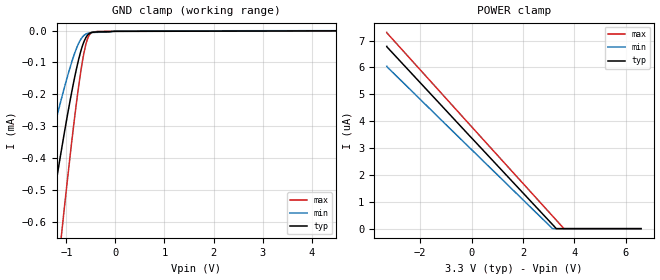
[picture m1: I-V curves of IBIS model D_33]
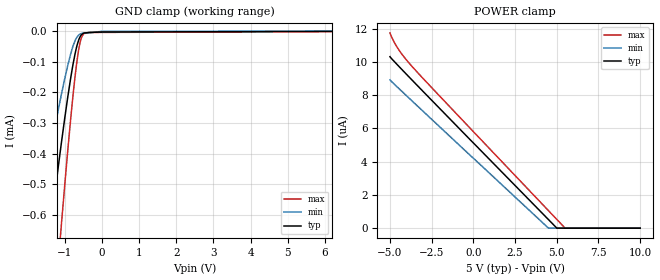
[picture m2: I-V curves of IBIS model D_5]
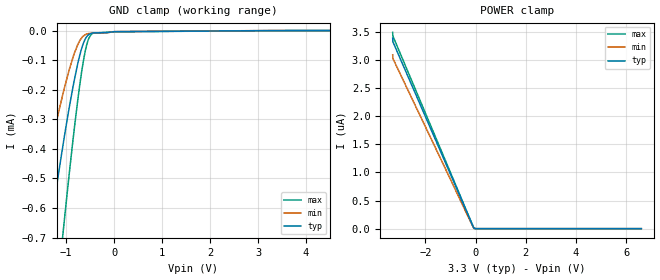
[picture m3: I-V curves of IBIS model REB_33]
| Texas Instruments Incorporated
| Isolated 5-V Full Duplex RS-485 Transceiver
| Bit Rate of 20 Mbps
| Marketing part#   Voltage Range   Package-type   #pins/pkg drawing
| ISO3086DW   3.15V - 5.5V   R-PSOP-G16   16-pin DW
[IBIS Ver]   4.1
[File name]   iso3086e.ibs
[File Rev]   1.0
[Date]   05/04/2010
[Source]   Model built from TISPICE simulations at:
   Texas Instruments Incorporated.
   Analog-eLab, HPA
   12500 TI Blvd
   Dallas, TX -75243
   For Support e-mail: elab_scm_ibis@list.ti.com
[Notes]   Revision History
   Rev 1.0: 05/04/2010
   - Model based on simulations from TIspice
   - Based on simulations, C_comp_typ was lower that C_comp_min
   for pins R, Y and Z
[Disclaimer] This product is designed as an aid for customers of Texas
   Instruments.
   No warranties, either expressed or implied, with respect
   to this third party software (if any) or with respect to
   its fitness for any particular purpose is claimed by Texas
   Instruments or the author. The software (if any) is provided
   solely on an "as is" basis. The entire risk as to its quality
   and performance is with the customer
[Copyright]   (C)Copyright 2010 Texas Instruments Incorporated.
   All rights reserved.
|   Component iso3086e
[Component]   iso3086e
[Manufacturer]  Texas Instruments Incorporated
[Package]   |16-pin PSOP DW package
|   typ   min   max
R_pkg   0.004632   0.00255   0.00893
L_pkg   1.232951nH   0.61490nH   2.36061nH
C_pkg   0.306389pF   0.17825pF   0.45943pF
[Pin] signal_name   model_name   R_pin   L_pin   C_pin
   1  Vcc1   POWER   0.00876   2.29508nH   0.42042pF
   2  GND1   GND   0.00503   1.29566nH   0.28670pF
   3  R   R   0.00282   0.68474nH   0.18911pF
   4  REB   REB   0.00255   0.61553nH   0.17825pF
   5  DE   DE   0.00255   0.61490nH   0.17895pF
   6  D   D   0.00282   0.68226nH   0.19223pF
   7  GND1   GND   0.00276   0.68705nH   0.18198pF
   8  GND1   GND   0.00827   2.24969nH   0.38663pF
   9  GND2   GND   0.00893   2.36061nH   0.43538pF
   10  GND2   GND   0.00586   1.55263nH   0.35752pF
   11  Y   Y   0.00289   0.70650nH   0.19678pF
   12  Z   Z   0.00255   0.61510nH   0.17846pF
   13  B   B   0.00255   0.61510nH   0.17846pF
   14  A   A   0.00289   0.70650nH   0.19678pF
   15  GND2   GND   0.00622   1.64583nH   0.37990pF
   16  Vcc2   POWER   0.00858   2.25489nH   0.45943pF
[Diff_pin]   inv_pin   vdiff   tdelay_typ   tdelay_min   tdelay_max
| The A and B are Diff_pins
| The Y and X are Diff_pins
11   12   0.9   NA   NA   NA
13   14   0.9   NA   NA   NA
[series pin mapping]  pin_2   model_name
4   7   series1M   |REB
5   1   series1M   |DE
6   7   series1M   |D
[Pin Mapping]pulldown_ref pullup_ref gnd_clamp_ref power_clamp_ref |ext_ref
1   NC   PWRBUS1  |Vcc1
2   GNDBUS1   NC   |GND1
3   GNDBUS1   PWRBUS1   NC   NC   | R
4   NC   NC   GNDBUS1   PWRBUS1  | RE_N
5   NC   NC   GNDBUS1   PWRBUS1  | DE
6   NC   NC   GNDBUS1   PWRBUS1  | D
7   GNDBUS1   NC   |GND1
8   GNDBUS1   NC   |GND1
9   GNDBUS2   NC   |GND2 to Y/Z
10   GNDBUS2   NC   |GND2 to Y/Z
11   GNDBUS2   PWRBUS2   NC   NC   | Y   Diff. Out. P
12   GNDBUS2   PWRBUS2   NC   NC   | Z   Diff. Out. N
13   NC   NC   GNDBUS2   PWRBUS2  | B   Diff. Inp. N
14   NC   NC   GNDBUS2   PWRBUS2  | A   Diff. Inp. P
15   GNDBUS2   NC   |GND2 to Y/Z
16   NC   PWRBUS2  |VCC2 to Y/Z
[Model Selector] series1M
series1M_33   series1M model for 3.15V  - 3.60V
series1M_5   series1M model for 4.50V  - 5.50V
[Model Selector] D
D_33   D Input model for 3.15V  - 3.60V
D_5   D Input model for 4.50V  - 5.50V
[Model Selector] DE
DE_33   DE Input model for 3.15V  - 3.60V
DE_5   DE Input model for 4.50V  - 5.50V
[Model Selector] REB
REB_33   REB Input model for 3.15V  - 3.60V
REB_5   REB Input model for 4.50V  - 5.50V
[Model Selector] R
R_33   R Output model for 3.15V  - 3.60V
R_5   R Output model for 4.50V  - 5.50V
[Model Selector] A
A_33   A Differential Input model for 3.15V  - 3.60V  |positive pin
A_5   A Differential Input model for 4.50V  - 5.50V
[Model Selector] B
B_33   B Differential Input model for 3.15V  - 3.60V  |negative pin
B_5   B Differential Input model for 4.50V  - 5.50V
[Model Selector] Y
Y_33   Y Differential 3-state model for 3.15V  - 3.60V  |positive pin
Y_5   Y Differential 3-state model for 4.50V  - 5.50V
[Model Selector] Z
Z_33   Z Differential 3-state model for 3.15V  - 3.60V  |negative pin
Z_5   Z Differential 3-state model for 4.50V  - 5.50V
|   series1M_33 Model
[Model]   series1M_33
Model_type   Series
C_comp   0pF   0pF   0pF
[Voltage Range]   3.3V   3.15V   3.6V
[Pullup Reference]   3.3V   3.15V   3.6V
|It is pullup   resistor for D and REB
|It is pulldown resistor for DE
[Temperature Range]   40   125   -40
[R series]   1e6   NA   NA
|   series1M_5 Model
[Model]   series1M_5
Model_type   Series
C_comp   0pF   0pF   0pF
[Voltage Range]   5V   4.5V   5.5V
[Pullup Reference]   5V   4.5V   5.5V
|It is pullup   resistor for D and REB
|It is pulldown resistor for DE
[Temperature Range]   40   125   -40
[R series]   1e6   NA   NA
| Models and submodels in the file (18): series1M_33 (Series), series1M_5 (Series), D_33 (Input), D_5 (Input), DE_33 (Input), DE_5 (Input), REB_33 (Input), REB_5 (Input), R_33 (3-state), R_5 (3-state), A_33 (Input), B_33 (Input), A_5 (Input), B_5 (Input), Y_33 (3-state), Z_33 (3-state), Y_5 (3-state), Z_5 (3-state)
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|   D_33 Model
[Model]   D_33
Model_type   Input
Vinl   = 0.8
Vinh   = 2
|   typ   min   max
C_comp   768fF   754fF   769fF
[Voltage Range]   3.3   3.15   3.6
[Temperature Range]   40   125   -40
[Power Clamp Reference]   3.3   3.15   3.6
[GND Clamp Reference]   0   0   0
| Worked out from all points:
|   GND clamp passes 1 mA (typ) near -1.74 V on its own axis
[GND Clamp]
|   Voltage   I(typ)   I(min)   I(max)
-3.3V     -2.774mA   -1.822mA   -4.341mA
-1.741V   -1.005mA   -627.4uA   -1.627mA
-1.419V   -681.4uA   -413.7uA   -1.123mA
-1.345V   -608.1uA   -365.7uA   -1.009mA
-1.127V   -399.6uA   -230.1uA   -682.4uA
-1.048V   -327.3uA   -183.6uA   -567.2uA
-800.3mV  -124.8uA   -58.6uA    -234.5uA
-671.5mV  -47.79uA   -20.16uA   -95.83uA
-572.6mV  -15.26uA   -8.85uA    -27.84uA
-488.4mV  -6.178uA   -6.221uA   -6.699uA
-354.8mV  -3.975uA   -5.385uA   -2.478uA
6.6V      0A         0A         0A
[POWER Clamp]
|   Voltage   I(typ)   I(min)   I(max)
-3.3V     6.784uA    6.046uA    7.304uA
3.155V    152nA      0A         469.9nA
3.303V    0A         0A         313.2nA
3.6V      0A         0A         0A
6.6V      0A         0A         0A
|   D_5 Model
[Model]   D_5
Model_type   Input
Vinl   = 0.8
Vinh   = 2
|   typ   min   max
C_comp   719fF   718fF   752fF
[Voltage Range]   5   4.5   5.5
[Temperature Range]   40   125   -40
[Power Clamp Reference]   5   4.5   5.5
[GND Clamp Reference]   0   0   0
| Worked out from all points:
|   GND clamp passes 1 mA (typ) near -1.73 V on its own axis
[GND Clamp]
|   Voltage   I(typ)   I(min)   I(max)
-5V       -4.946mA   -3.314mA   -7.567mA
-1.812V   -1.082mA   -677.1uA   -1.752mA
-1.685V   -951.3uA   -590.3uA   -1.547mA
-1.445V   -709.6uA   -431.2uA   -1.172mA
-1.355V   -620.4uA   -372.8uA   -1.034mA
-1.1V     -376.7uA   -214.4uA   -650.4uA
-912.5mV  -212.6uA   -110.4uA   -385.3uA
-770mV    -105.6uA   -47.46uA   -204.5uA
-665mV    -46uA      -19.19uA   -94.93uA
-560mV    -13.91uA   -8.401uA   -26.09uA
-350mV    -4.646uA   -5.549uA   -4.688uA
10V       0A         0A         0A
[POWER Clamp]
|   Voltage   I(typ)   I(min)   I(max)
-5V       10.32uA    8.921uA    11.74uA
-4.782V   10.06uA    8.696uA    11.25uA
-4.482V   9.745uA    8.411uA    10.74uA
-4.122V   9.367uA    8.07uA     10.25uA
-3.62V    8.845uA    7.596uA    9.659uA
4.503V    514.4nA    0A         1.052uA
5.005V    0A         0A         522.2nA
5.5V      0A         0A         0A
10V       0A         0A         0A
|   REB_33 Model
[Model]   REB_33
Model_type   Input
Vinl   = 0.8
Vinh   = 2
|   typ   min   max
C_comp   5.79pF   5.78pF   5.79pF
[Voltage Range]   3.3   3.15   3.6
[Temperature Range]   40   125   -40
[Power Clamp Reference]   3.3   3.15   3.6
[GND Clamp Reference]   0   0   0
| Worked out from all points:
|   GND clamp passes 1 mA (typ) near -1.61 V on its own axis
[GND Clamp]
|   Voltage   I(typ)   I(min)   I(max)
-3.3V     -3.18mA    -2.151mA   -4.772mA
-1.676V   -1.075mA   -676.4uA   -1.73mA
-1.335V   -676.9uA   -405.7uA   -1.132mA
-1.058V   -379.6uA   -208.5uA   -673.8uA
-924mV    -250uA     -126.3uA   -467.7uA
-755.7mV  -110.5uA   -46.71uA   -233uA
-666.6mV  -55.52uA   -22.65uA   -129.1uA
-587.4mV  -24.64uA   -12.83uA   -58.94uA
-528mV    -13.46uA   -9.998uA   -26.57uA
-468.6mV  -9.118uA   -8.887uA   -11.88uA
1.65mV    -3.737uA   -3.472uA   -3.985uA
6.6V      0A         0A         0A
[POWER Clamp]
|   Voltage   I(typ)   I(min)   I(max)
-3.3V     3.392uA    3.093uA    3.493uA
-3.295V   3.328uA    3.03uA     3.429uA
-67.65mV  8.615nA    3.584nA    9.353nA
6.6V      0A         0A         0A
